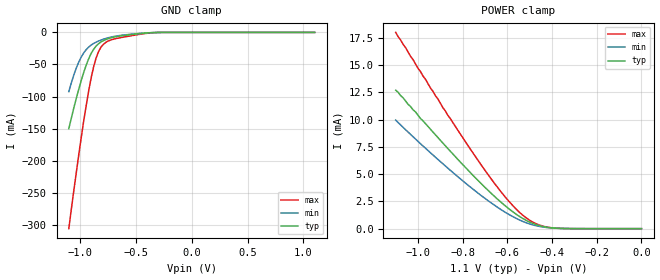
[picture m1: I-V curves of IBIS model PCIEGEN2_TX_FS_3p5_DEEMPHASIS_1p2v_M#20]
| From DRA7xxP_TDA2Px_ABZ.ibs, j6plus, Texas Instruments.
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| Model based on original model for USB3_PCIEGEN1_PCIEGEN2_TX
|   Sub model PCIEGEN2_TX_FS_3p5_DEEMPHASIS_1p2v
[model]   PCIEGEN2_TX_FS_3p5_DEEMPHASIS_1p2v_M#20
|[Description]  [1.1V-3-STATE-X-X]
|   , ,
|[Input Load]
|[Output Drive]
|Voltage   1.1V
|Mode   3-STATE
Model_type   3-state
Polarity   Non-Inverting
Enable   Active-Low
Cref =  15.0000pF
Rref =  100.0000M
Vref =  0V
Vmeas =  0.55
C_comp   0.4p   0.4p   0.4p
[Temperature Range]   25   125   -40
[Voltage Range]   1.1   1.078   1.122
[Driver Schedule]
DRIVER_LVL0   NA   200ps   NA   200ps
DRIVER_LVL1   NA   200ps   NA   200ps
DRIVER_LVL2   0ps   NA   0ps   NA
DRIVER_LVL3   0ps   NA   0ps   NA
DRIVER_LVL4   NA   200ps   NA   200ps
DRIVER_LVL5   0ps   NA   0ps   NA
DRIVER_LVL6   0ps   NA   0ps   NA
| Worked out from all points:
|   GND clamp passes 1 mA (typ) near -0.41 V on its own axis
|   POWER clamp passes 1 mA (typ) near -0.54 V on its own axis
[POWER_clamp]
-1.1V     12.7mA     9.96mA     18mA
-966.7mV  9.63mA     7.38mA     13.7mA
-944.4mV  9.12mA     6.96mA     12.9mA
-911.1mV  8.36mA     6.35mA     11.9mA
-888.9mV  7.85mA     5.95mA     11.1mA
-711.1mV  4mA        2.94mA     5.66mA
-611.1mV  2.12mA     1.52mA     2.94mA
-533.3mV  961uA      684uA      1.27mA
-500mV    598uA      429uA      765uA
-466.7mV  333uA      246uA      410uA
-400mV    69.4uA     61.7uA     78uA
0V        120nA      895nA      288nA
[Pulldown]
-1.1V     0A         0A         0A
-1.067V   0A         0A         0A
-1.033V   0A         0A         0A
2.2V      0A         0A         0A
[Pullup]
-1.1V     0A         0A         0A
-1.067V   0A         0A         0A
-1.033V   0A         0A         0A
2.2V      0A         0A         0A
[GND_clamp]
-1.1V     -150mA     -92.3mA    -306mA
-1.056V   -118mA     -66.6mA    -247mA
-1.011V   -88.7mA    -46.3mA    -191mA
-966.7mV  -62.4mA    -32mA      -138mA
-922.2mV  -41.1mA    -22.9mA    -91.2mA
-877.8mV  -26.3mA    -17.2mA    -53.6mA
-855.6mV  -21.3mA    -15.2mA    -39.8mA
-833.3mV  -17.6mA    -13.4mA    -29.7mA
-788.9mV  -12.7mA    -10.5mA    -18.3mA
-677.8mV  -6.75mA    -5.74mA    -9.67mA
-322.2mV  -147uA     -254uA     -266uA
1.1V      120nA      909nA      272nA
[Ramp]
dV/dt_f 55m/24.496914p  54m/31.970054p  56m/18.193627p
dV/dt_r 55m/24.267571p  54m/32.968711p  56m/17.881799p
R_load = 50
